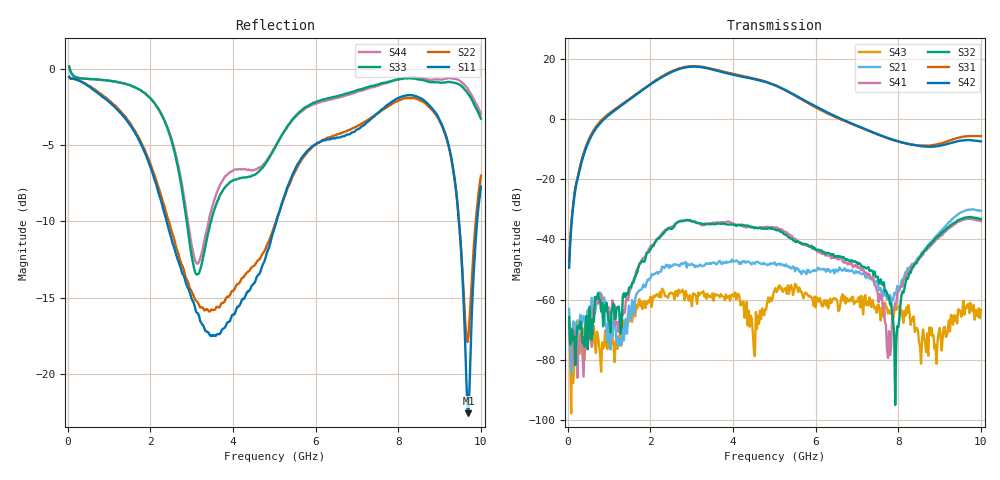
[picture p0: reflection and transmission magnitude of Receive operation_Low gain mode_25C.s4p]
! Device:  ADRF5545A
! Description: Dual-Channel, Receiver Front End
! Frequency:  2.4 -  4.2 GHz
! Ports:
!	ANT-CHA	= Port 1
!	ANT-CHB	= Port 2
!  RXOUT-CHA = Port 3
!	RXOUT-CHB = Port 4
! VDD1-CHA, VDD1-CHB, VDD2-CHA, VDD2-CHB, and SWVDD-CHAB = 5 V
! SWCTRL-CHAB = 0 V,  PD-CHAB = 0 V,BP-CHA=BP-CHB=5V
! Temp=25C
! Data:  Data was collected using a calibrated 4 port network analyzer and de-embedded using AtaiTec's In Situ De-Embedding.
! Note:  Analog Devices supplies this data as a sample of measured data
!  for this product.  Your particular data for this product may vary.
!  Data was taken at 25 degrees C.
!  Analog Devices reserves the right to change this data at anytime.
!Correction: S11(Full 4 Port(1,2,3,4))
!S12(Full 4 Port(1,2,3,4))
!S13(Full 4 Port(1,2,3,4))
!S14(Full 4 Port(1,2,3,4))
!S21(Full 4 Port(1,2,3,4))
!S22(Full 4 Port(1,2,3,4))
!S23(Full 4 Port(1,2,3,4))
!S24(Full 4 Port(1,2,3,4))
!S31(Full 4 Port(1,2,3,4))
!S32(Full 4 Port(1,2,3,4))
!S33(Full 4 Port(1,2,3,4))
!S34(Full 4 Port(1,2,3,4))
!S41(Full 4 Port(1,2,3,4))
!S42(Full 4 Port(1,2,3,4))
!S43(Full 4 Port(1,2,3,4))
!S44(Full 4 Port(1,2,3,4))
!S4P File: Measurements: <S11,S12,S13,S14>,
!<S21,S22,S23,S24>,
!<S31,S32,S33,S34>,
!<S41,S42,S43,S44>:
# Hz S  dB  R 50
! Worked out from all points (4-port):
!   400 points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, 34.98 MHz to 10 GHz, reference 50 ohm
!   strongest paths, dB at 34.98 MHz, 2.532 GHz, 5.03 GHz, 7.527 GHz, 10 GHz:
!     S42: -49.4, 15.7, 11.1, -5.2, -7.5
!     S31: -47.3, 15.9, 11.2, -5.3, -5.7
!     S32: -65.8, -36.4, -36.8, -54.0, -33.2
!     S41: -70.6, -35.6, -36.0, -60.8, -33.9
!     S21: -63.1, -48.9, -48.2, -56.4, -30.5
!     S43: -68.3, -58.0, -56.1, -61.7, -63.4
!   lowest |S11| = -22.6 dB at 9.7 GHz (marker M1), VSWR 1.16, Z = 43.4 + j2.16 ohm
!   |S11| at or under -10 dB: 2.396 GHz to 5.053 GHz (2.657 GHz wide, 71.3 % of centre); 9.47 GHz to 9.909 GHz (438.7 MHz wide, 4.53 % of centre)
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3.4975e7  -0.48 -10.3  -75.76 98.2  -68.57 -77.7  -66.99 -27.8
          -63.07 -41.7  -0.53 -10.2  -60.14 107.2  -65.75 -120.5
          -47.31 8.9  -65.78 -75.8  0.17 -6.6  -78.78 93.4
          -70.60 124.2  -49.41 -0.1  -68.32 -73.3  0.20 -6.6
2.182825e9  -7.96 -155.2  -51.15 97.8  -44.20 122.0  -74.97 128.5
            -51.43 97.7  -7.65 -155.0  -83.90 -133.2  -44.42 122.6
            13.30 140.9  -39.84 64.7  -2.54 -101.6  -60.50 149.2
            -39.66 69.6  13.08 142.7  -58.73 155.0  -2.56 -103.6
2.75725e9  -13.28 121.1  -49.36 60.8  -37.09 66.0  -68.69 113.8
           -47.89 58.6  -12.82 125.9  -70.98 75.4  -37.46 68.7
           17.03 73.9  -33.75 -19.6  -7.76 -131.2  -57.32 101.1
           -34.02 -18.8  16.83 76.3  -57.38 112.4  -7.42 -134.6
3.281725e9  -16.82 36.7  -47.86 45.8  -34.34 9.6  -72.62 109.5
            -48.83 39.4  -15.70 38.5  -71.12 85.6  -34.74 11.7
            17.27 9.0  -34.87 -83.8  -12.30 -85.7  -55.50 85.2
            -35.27 -79.6  17.10 11.2  -57.16 78.5  -11.63 -90.9
4.95505e9  -10.88 40.3  -46.34 -16.7  -34.16 -130.1  -66.19 -7.4
           -48.02 -8.1  -10.66 42.8  -69.92 59.8  -34.39 -125.4
           11.59 -150.7  -36.48 125.7  -5.46 166.2  -61.71 92.1
           -35.97 125.9  11.52 -146.9  -59.81 112.8  -5.39 172.0
9.7003e9  -22.60 160.5  -30.57 -126.0  -43.04 55.9  -57.08 51.2
          -30.19 -127.8  -17.48 158.8  -57.84 39.6  -43.71 56.1
          -5.68 -27.2  -32.60 -91.9  -1.65 103.9  -62.33 33.8
          -33.14 -92.2  -6.99 -26.7  -61.43 14.9  -1.36 98.4
1e10  -7.71 -145.5  -31.02 -176.2  -43.01 32.5  -54.90 68.6
      -30.53 -178.8  -7.00 -157.8  -58.95 74.1  -44.26 28.5
      -5.69 -59.4  -33.23 -148.0  -3.24 102.1  -59.50 41.3
      -33.93 -146.8  -7.45 -57.4  -63.38 32.8  -2.93 98.6
